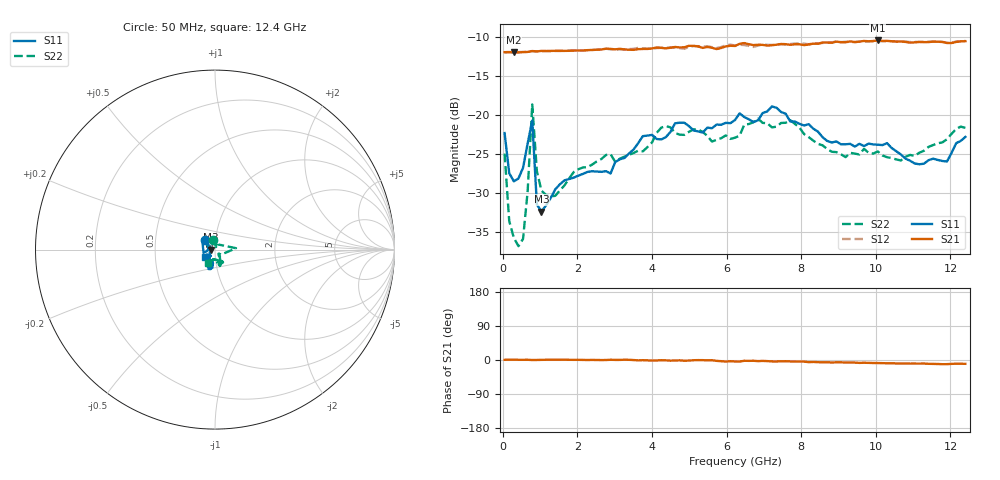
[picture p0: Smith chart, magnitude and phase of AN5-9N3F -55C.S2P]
! Network Analyzer HP8720D.06.14 Serial No. US36140669
! 24 Jul 2008  14:36:04
! Frequency  S11  S21  S12  S22
# HZ  S  DB R 50
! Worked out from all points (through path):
!   101 points, 50 MHz to 12.4 GHz, reference 50 ohm
!   highest |S21| = -10.40 dB at 10.05 GHz (marker M1); lowest = -11.9 dB at 297 MHz (marker M2)
!   group delay of S21, straight-line fit = 2.83 ps
!   lowest |S11| = -32.3 dB at 1.038 GHz (marker M3), VSWR 1.05, Z = 47.6 - j0.047 ohm
!   |S11| at or under -10 dB: start of sweep to end of sweep
!   |S22| runs from -36.8 to -18.6 dB; largest |S21 - S12| = 0.0091
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5e7  -22.27 134.4  -11.89 0.5  -11.95 0.5  -24.90 100.8
1.735e8  -27.41 159.5  -11.88 0.8  -11.91 0.5  -33.55 78.7
2.97e8  -28.46 172.3  -11.93 1.0  -11.92 0.6  -35.70 67.8
5.44e8  -26.73 -169.6  -11.89 0.5  -11.87 0.5  -35.84 79.4
6.675e8  -23.59 -164.0  -11.87 0.6  -11.86 0.6  -29.75 91.6
7.91e8  -20.66 140.8  -11.76 -0.0  -11.75 0.1  -18.60 3.8
9.145e8  -31.43 149.8  -11.80 0.1  -11.80 0.4  -27.15 -39.6
1.038e9  -32.34 -178.8  -11.74 0.4  -11.77 0.6  -29.67 -44.3
1.4085e9  -29.48 -151.7  -11.72 0.6  -11.75 0.5  -30.32 -50.9
2.1495e9  -27.51 -130.5  -11.69 0.2  -11.67 0.4  -26.68 -53.7
2.8905e9  -27.45 -125.2  -11.48 0.6  -11.53 0.6  -24.98 -61.0
3.755e9  -22.66 -121.1  -11.49 -0.5  -11.40 0.2  -24.62 -64.1
4.249e9  -23.09 -116.0  -11.34 -0.5  -11.34 -0.7  -21.58 -64.3
6.225e9  -20.60 -112.8  -11.11 -3.8  -11.04 -2.2  -22.86 -74.9
6.8425e9  -20.64 -113.0  -10.95 -3.0  -11.06 -4.3  -20.43 -74.0
7.213e9  -18.86 -108.5  -11.01 -3.8  -10.97 -3.5  -21.54 -72.0
7.707e9  -20.79 -98.4  -10.95 -3.8  -10.85 -4.8  -20.62 -72.5
8.3245e9  -21.71 -99.2  -10.80 -5.1  -10.79 -4.9  -23.24 -68.8
1.00535e10  -23.77 -124.5  -10.40 -8.1  -10.50 -8.6  -24.63 -99.9
1.0424e10  -24.19 -124.2  -10.50 -8.5  -10.49 -9.1  -25.48 -100.7
1.1906e10  -25.91 -143.2  -10.72 -11.0  -10.69 -11.0  -23.07 -118.2
1.24e10  -22.77 -142.8  -10.49 -10.1  -10.45 -10.1  -21.60 -118.0
